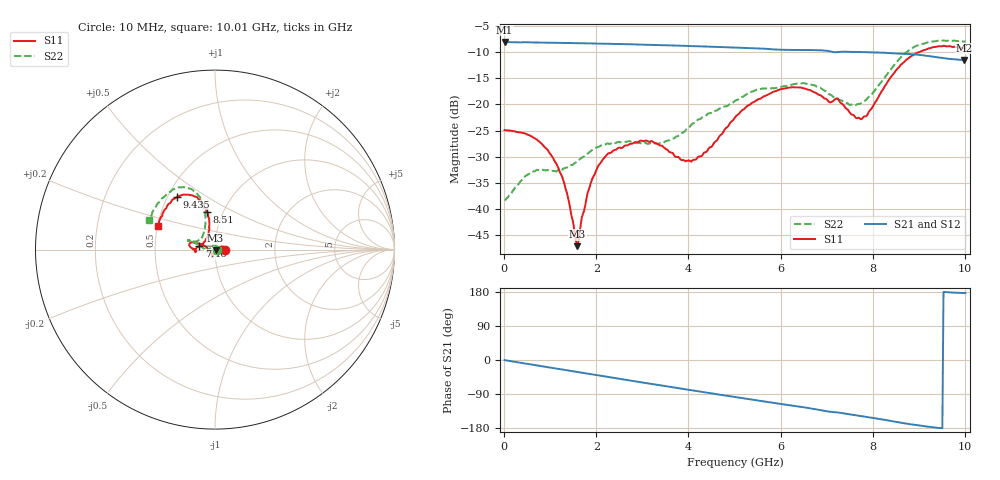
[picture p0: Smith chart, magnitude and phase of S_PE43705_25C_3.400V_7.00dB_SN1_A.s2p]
! Device ID: PE43705
! Serial: 1
! Insertion: A
! Impedance: 50 ohm
! Temp: 25C
! VDD: 3.400V
! Attenuation Step: 7.00dB
#  Hz  S  RI  R  50
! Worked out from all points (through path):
!   401 points, 10 MHz to 10.01 GHz, reference 50 ohm
!   highest |S21| = -8.02 dB at 10 MHz (marker M1); lowest = -11.5 dB at 9.985 GHz (marker M2)
!   group delay of S21, straight-line fit = 52.3 ps
!   lowest |S11| = -47.2 dB at 1.585 GHz (marker M3), VSWR 1.01, Z = 50.3 - j0.328 ohm
!   |S11| at or under -10 dB: start of sweep to 8.996 GHz
!   |S22| runs from -38.3 to -7.7 dB; largest |S21 - S12| = 0.0034
!   S11 on the Smith chart (normalised r, x): 10 MHz: 1.12, +0.00; 7.46 GHz: 0.84, +0.04; 8.51 GHz: 0.84, +0.37; 9.435 GHz: 0.56, +0.38; 10.01 GHz: 0.50, +0.15
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1e7  0.0568 1.96e-05  0.3973 -0.00191  0.3977 -0.0017  0.0122 0.00031
5.35e8  0.0484 0.016  0.3866 -0.0752  0.3867 -0.0749  0.00768 0.02
1.01e9  0.0295 0.0154  0.3664 -0.1367  0.3664 -0.1363  -0.00673 0.0219
1.31e9  0.0156 0.0073  0.349 -0.1723  0.3491 -0.1721  -0.0181 0.0164
1.585e9  0.00292 -0.00326  0.3293 -0.2035  0.3295 -0.2034  -0.0271 0.00809
1.685e9  -0.000529 -0.00826  0.3217 -0.2144  0.3218 -0.2143  -0.0306 0.00473
1.885e9  -0.00768 -0.0162  0.3053 -0.2351  0.3054 -0.2347  -0.0359 -0.00155
2.21e9  -0.0135 -0.0292  0.2754 -0.2657  0.2755 -0.2655  -0.0403 -0.0102
2.935e9  -0.0167 -0.0412  0.1982 -0.3193  0.1988 -0.3194  -0.0411 -0.0121
3.36e9  -0.0144 -0.0384  0.1493 -0.3396  0.1497 -0.3392  -0.0407 -0.0106
4.11e9  -0.027 -0.0119  0.0593 -0.3583  0.0598 -0.3581  -0.0659 0.0073
5.01e9  -0.07 0.0272  -0.0468 -0.3481  -0.0463 -0.3483  -0.1032 0.033
5.935e9  -0.1306 0.0403  -0.1404 -0.305  -0.1392 -0.3057  -0.1353 0.0518
6.685e9  -0.1334 0.011  -0.2066 -0.2601  -0.2065 -0.2603  -0.1451 0.0501
7.46e9  -0.0864 0.0211  -0.2547 -0.1943  -0.254 -0.1948  -0.0865 0.0548
7.81e9  -0.0518 0.0565  -0.2729 -0.1632  -0.2727 -0.1636  -0.0674 0.0849
8.36e9  -0.0331 0.1714  -0.2931 -0.1056  -0.292 -0.107  -0.0562 0.2017
8.51e9  -0.0442 0.2086  -0.2953 -0.0874  -0.294 -0.0894  -0.0656 0.2426
8.91e9  -0.0965 0.2885  -0.2993 -0.0472  -0.2971 -0.0474  -0.1286 0.3353
9.435e9  -0.21 0.295  -0.2816 -0.00408  -0.2813 -0.00363  -0.24 0.3298
9.985e9  -0.3129 0.1414  -0.2668 0.0155  -0.2675 0.0146  -0.3589 0.1776
1.001e10  -0.3201 0.1319  -0.2678 0.0157  -0.2689 0.0149  -0.3666 0.1664
